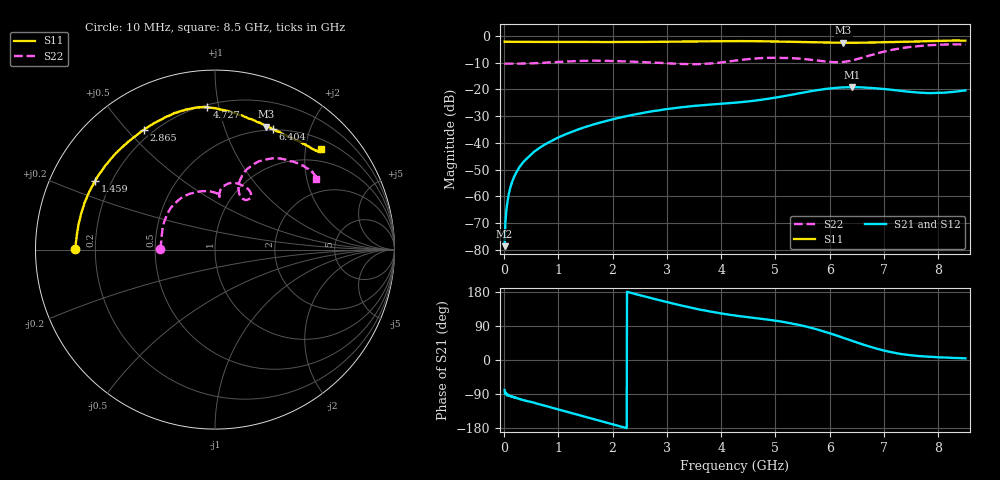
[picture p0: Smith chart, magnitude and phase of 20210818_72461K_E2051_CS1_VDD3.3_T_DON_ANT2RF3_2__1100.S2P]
!Agilent Technologies,E5071C,MY46417908,A.11.23
!Date: Wed Aug 18 14:29:34 2021
!Data & Calibration Information:
!Freq	S11:SOLT2(ON)	S21:SOLT2(ON)	S12:SOLT2(ON)	S22:SOLT2(ON)
!PortZ  Port1:50+j0  Port2:50+j0
!Above PortZ is port z conversion or system Z0 setting when saving the data.
!When reading, reference impedance value at option line is always used.
# Hz S dB R 50
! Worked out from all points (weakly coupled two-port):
!   1601 points, 10 MHz to 8.5 GHz, reference 50 ohm
!   highest |S21| = -19.18 dB at 6.409 GHz (marker M1); lowest = -78.7 dB at 10 MHz (marker M2)
!   lowest |S11| = -2.6 dB at 6.25 GHz (marker M3), VSWR 6.79, Z = 22.9 + j70.1 ohm
!   |S11| at or under -10 dB: nowhere
!   |S22| runs from -10.6 to -3.2 dB; largest |S21 - S12| = 0.00056
!   S11 on the Smith chart (normalised r, x): 10 MHz: 0.12, +0.00; 1.459 GHz: 0.14, +0.26; 2.865 GHz: 0.17, +0.56; 4.727 GHz: 0.22, +0.92; 6.404 GHz: 0.49, +1.48; 8.5 GHz: 0.70, +2.33
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1e7  -2.16 179.7  -78.65 -79.0  -79.53 -94.4  -10.35 179.5
6.30625e7  -2.20 178.6  -62.08 -91.3  -61.92 -92.5  -10.38 177.9
1.055125e8  -2.20 177.7  -57.61 -94.5  -57.67 -94.2  -10.38 176.6
1.798e8  -2.21 176.2  -52.97 -98.2  -53.08 -98.5  -10.40 174.3
3.018438e8  -2.23 173.7  -48.62 -103.8  -48.55 -103.7  -10.37 171.0
7.157312e8  -2.25 165.2  -41.05 -119.3  -41.05 -119.2  -10.05 158.6
1.426769e9  -2.27 151.0  -34.56 -147.2  -34.57 -147.2  -9.36 132.2
1.458606e9  -2.27 150.3  -34.33 -148.5  -34.34 -148.4  -9.35 131.0
2.1325e9  -2.28 136.3  -30.57 -174.9  -30.58 -175.0  -9.49 106.0
2.843538e9  -2.20 121.3  -27.85 158.5  -27.85 158.4  -10.06 88.2
2.864762e9  -2.20 120.9  -27.79 157.7  -27.78 157.6  -10.08 87.9
3.5758e9  -2.05 108.0  -26.07 134.0  -26.06 134.0  -10.58 85.0
4.255e9  -1.97 98.6  -24.98 117.3  -24.99 117.3  -9.26 83.8
4.727256e9  -2.01 93.0  -23.92 109.0  -23.92 109.0  -8.33 75.7
5.671769e9  -2.36 78.6  -20.63 84.4  -20.65 84.6  -8.98 55.6
6.25015e9  -2.58 67.3  -19.29 58.5  -19.31 58.5  -9.73 64.0
6.404031e9  -2.56 64.2  -19.19 50.9  -19.21 50.8  -9.21 67.3
6.409338e9  -2.54 64.1  -19.18 50.7  -19.20 50.5  -9.17 67.5
7.088538e9  -2.32 51.5  -20.05 22.1  -20.07 21.9  -5.47 64.9
7.491812e9  -2.16 46.1  -20.95 12.7  -20.96 12.5  -4.13 54.8
8.001212e9  -1.85 42.4  -21.33 7.1  -21.30 7.1  -3.30 41.4
8.5e9  -1.78 43.5  -20.41 4.3  -20.41 4.0  -3.29 34.8
